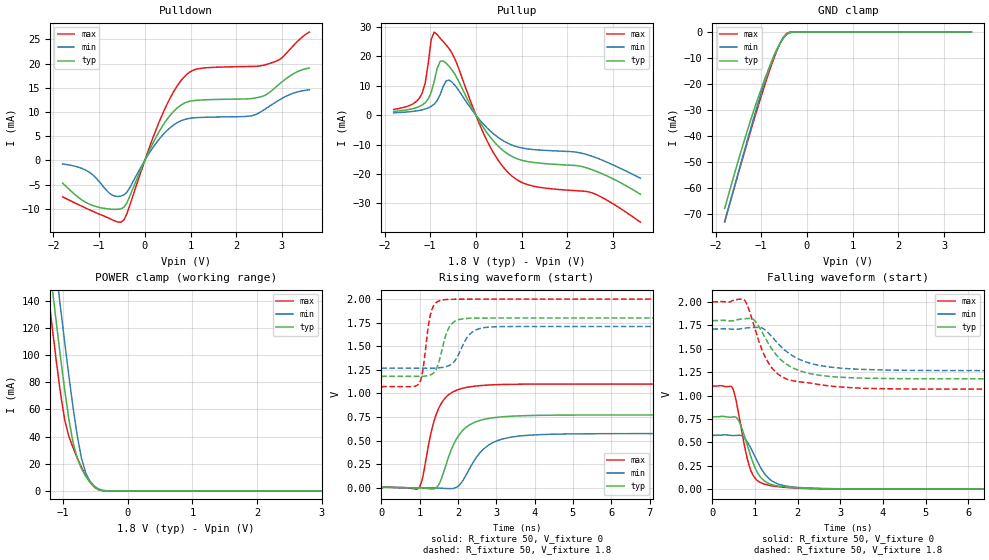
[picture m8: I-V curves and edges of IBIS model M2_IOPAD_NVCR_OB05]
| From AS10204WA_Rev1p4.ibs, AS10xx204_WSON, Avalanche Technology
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[Model] M2_IOPAD_NVCR_OB05
Model_type I/O
Enable   Active-High
Vinl  =  0.54
Vinh  =  1.26
Vmeas =  0.9
Cref  =  30e-12
| Capacitance  typ   min   max
C_comp   3.869840e-12   3.575244e-12   4.208825e-12
| Variables   typ   min   max
[GND Clamp Reference]   0   0   0
[POWER Clamp Reference]   1.8   1.71   2
[Pulldown Reference]   0   0   0
[Pullup Reference]   1.8   1.71   2
[Temperature Range]   25   105   -40
[Voltage Range]   1.8   1.71   2
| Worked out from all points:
|   slope of the pulldown table from 0 to 0.27 V, typ, clamps not added: 51.8 ohm
|   slope of the pullup table from 0 to 0.27 V, typ, clamps not added: 41.1 ohm
|   GND clamp passes 1 mA (typ) near -0.46 V on its own axis
|   POWER clamp passes 1 mA (typ) near -0.44 V on its own axis
|   falling waveform, R_fixture 50, V_fixture 0: 20-80 % time 370ps typ, 446ps min, 301ps max; typ from 0.772 V to 0 V
|   falling waveform, R_fixture 50, V_fixture 1.8: 20-80 % time 687ps typ, 815ps min, 547ps max; typ from 1.8 V to 1.18 V
|   rising waveform, R_fixture 50, V_fixture 0: 20-80 % time 530ps typ, 643ps min, 413ps max; typ from 0 V to 0.772 V
|   rising waveform, R_fixture 50, V_fixture 1.8: 20-80 % time 261ps typ, 359ps min, 184ps max; typ from 1.18 V to 1.8 V
[GND Clamp]
| Voltage   I(typ)   I(min)   I(max)
-1.8V     -67.84mA   -73.19mA   -72.81mA
-1.499V   -49.26mA   -53.93mA   -54.28mA
-1.303V   -37.87mA   -41.64mA   -42.4mA
-1.108V   -27.29mA   -29.68mA   -30.84mA
-912.4mV  -17.6mA    -18.46mA   -19.84mA
-782.1mV  -11.7mA    -11.87mA   -13.01mA
-651.7mV  -6.447mA   -6.494mA   -6.896mA
-521.4mV  -2.255mA   -2.526mA   -2.141mA
-456.2mV  -849.3uA   -1.156mA   -679.4uA
-391mV    -172uA     -356.5uA   -88.88uA
-260.7mV  -2.088uA   -12.98uA   -254.3nA
3.6V      0A         0A         0A
[POWER Clamp]
| Voltage   I(typ)   I(min)   I(max)
-1.8V     419.8mA    456.6mA    390.9mA
-1.238V   178mA      215.7mA    148.4mA
-1.173V   151mA      188.6mA    121.7mA
-1.108V   124.5mA    161.8mA    96mA
-1.043V   98.85mA    135.4mA    72.14mA
-977.6mV  74.56mA    109.6mA    52.56mA
-912.4mV  52.76mA    84.78mA    40.16mA
-847.2mV  35.48mA    61.36mA    31.71mA
-716.9mV  16.42mA    23.91mA    17.31mA
-651.7mV  10.9mA     13.27mA    11.28mA
-456.2mV  1.168mA    1.554mA    921.1uA
3.6V      0A         0A         0A
[Pulldown]
| Voltage   I(typ)   I(min)   I(max)
-1.8V     -4.699mA   -763.7uA   -7.55mA
-1.238V   -8.945mA   -2.323mA   -10.1mA
-782.1mV  -10.06mA   -6.741mA   -11.98mA
-521.4mV  -10.01mA   -7.379mA   -12.78mA
-391mV    -8.736mA   -6.551mA   -10.98mA
372.4mV   6.876mA    5.04mA     9.257mA
869mV     11.82mA    8.439mA    17.32mA
1.241V    12.47mA    8.871mA    19.03mA
2.352V    12.79mA    9.242mA    19.4mA
2.766V    14.31mA    11.43mA    20.12mA
3.248V    17.87mA    13.86mA    23.67mA
3.6V      19.07mA    14.57mA    26.49mA
[Pullup]
| Voltage   I(typ)   I(min)   I(max)
-1.8V     1.265mA    795.4uA    1.963mA
-1.173V   3.489mA    1.833mA    7.625mA
-1.108V   4.286mA    2.109mA    11.06mA
-977.6mV  7.759mA    3mA        25.76mA
-912.4mV  11.52mA    3.775mA    28.29mA
-782.1mV  18.3mA     7.007mA    26.2mA
-586.6mV  16.62mA    11.93mA    22.65mA
248.3mV   -6.114mA   -4.385mA   -8.852mA
744.8mV   -13.65mA   -9.886mA   -20.12mA
1.241V    -16.05mA   -11.68mA   -24.1mA
2.559V    -18.65mA   -14.06mA   -26.53mA
3.6V      -26.91mA   -21.45mA   -36.43mA
[Ramp]
dV/dt_r   0.463316/0.530243n  0.344907/0.643323n  0.66012/0.41274n
dV/dt_f   0.372865/0.686555n  0.266377/0.815444n  0.559402/0.546995n
R_load = 50
[Falling Waveform]
R_fixture = 50
V_fixture = 0
V_fixture_min = 0
V_fixture_max = 0
| Time   V(typ)   V(min)   V(max)
0s        772.2mV    574.8mV    1.1V
480.1ps   771mV      572.6mV    1.075V
545.6ps   770.1mV    573.6mV    969.9mV
639ps     712.4mV    576.6mV    745.7mV
823ps     464.3mV    502.1mV    318mV
970.5ps   264mV      376.7mV    136.6mV
1.21ns    91.22mV    174mV      55.35mV
1.59ns    29.99mV    48.44mV    23.79mV
3.646ns   1.033mV    1.612mV    643.1uV
21.88ns   194.5nV    541.1nV    178.6nV
[Falling Waveform]
R_fixture = 50
V_fixture = 1.8
V_fixture_min = 1.71
V_fixture_max = 2
| Time   V(typ)   V(min)   V(max)
0s        1.8V       1.71V      2V
748.5ps   1.821V     1.72V      2.023V
854.9ps   1.824V     1.725V     1.923V
976ps     1.808V     1.728V     1.748V
1.206ns   1.645V     1.712V     1.444V
1.547ns   1.41V      1.553V     1.227V
2.082ns   1.26V      1.378V     1.145V
2.869ns   1.2V       1.299V     1.097V
5.333ns   1.179V     1.267V     1.069V
21.88ns   1.179V     1.266V     1.068V
[Rising Waveform]
R_fixture = 50
V_fixture = 0
V_fixture_min = 0
V_fixture_max = 0
| Time   V(typ)   V(min)   V(max)
0s        71.62nV    371.8nV    128.3nV
964.7ps   -357uV     1.137mV    -7.097mV
1.081ns   -2.826mV   838.7uV    113.4mV
1.359ns   -11.16mV   -1.261mV   683.5mV
1.543ns   70.17mV    -3.767mV   879.7mV
1.949ns   510.1mV    3.549mV    1.032V
2.404ns   688.6mV    274.8mV    1.076V
2.988ns   745.6mV    493.6mV    1.093V
4.054ns   767.8mV    562.3mV    1.099V
21.88ns   772.2mV    574.8mV    1.1V
[Rising Waveform]
R_fixture = 50
V_fixture = 1.8
V_fixture_min = 1.71
V_fixture_max = 2
| Time   V(typ)   V(min)   V(max)
0s        1.178V     1.266V     1.068V
972.5ps   1.18V      1.267V     1.098V
1.075ns   1.181V     1.267V     1.227V
1.3ns     1.2V       1.267V     1.863V
1.465ns   1.287V     1.27V      1.972V
1.636ns   1.551V     1.279V     1.993V
1.923ns   1.766V     1.347V     1.998V
2.349ns   1.797V     1.643V     1.999V
2.873ns   1.799V     1.705V     2V
21.88ns   1.8V       1.71V      2V
